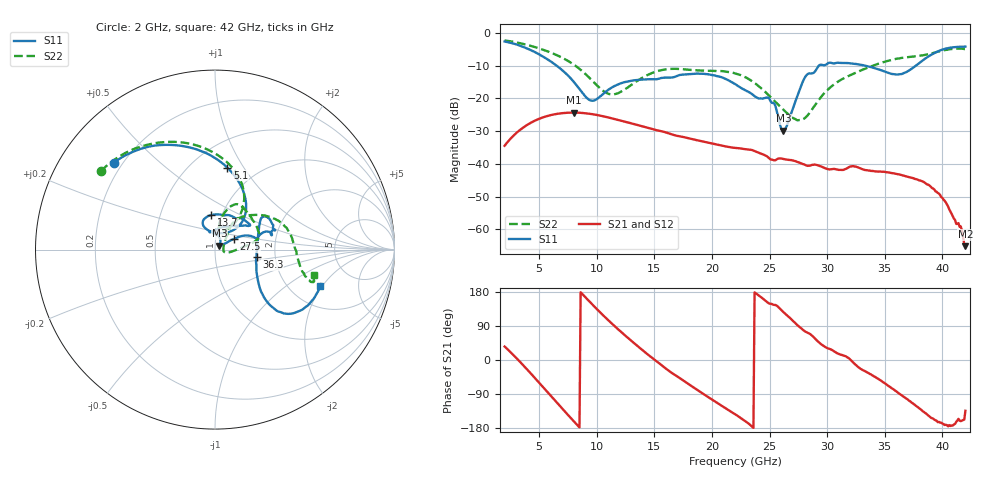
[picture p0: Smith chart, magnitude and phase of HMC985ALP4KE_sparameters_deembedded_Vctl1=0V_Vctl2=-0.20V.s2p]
!s2p File: Measurements: S11, S21, S12, S22
# GHz S dB R 50.0
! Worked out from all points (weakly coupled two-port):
!   401 points, 2 GHz to 42 GHz, reference 50 ohm
!   highest |S21| = -24.31 dB at 8 GHz (marker M1); lowest = -65.2 dB at 42 GHz (marker M2)
!   lowest |S11| = -29.8 dB at 26.2 GHz (marker M3), VSWR 1.07, Z = 52.5 + j2.21 ohm
!   |S11| at or under -10 dB: 6.529 GHz to 29.27 GHz (22.75 GHz wide, 127 % of centre); 33.34 GHz to 37.69 GHz (4.349 GHz wide, 12.2 % of centre)
!   |S22| runs from -26.7 to -2.3 dB; largest |S21 - S12| = 0.00014
!   S11 on the Smith chart (normalised r, x): 2 GHz: 0.17, +0.36; 5.1 GHz: 0.73, +0.85; 13.7 GHz: 0.89, +0.35; 27.5 GHz: 1.22, +0.15; 36.3 GHz: 1.60, -0.14; 42 GHz: 2.91, -1.91
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2  -2.57 139.4  -34.46 35.6  -34.48 35.6  -2.25 145.5
3.5  -4.07 111.5  -29.19 -10.1  -29.19 -10.1  -3.22 121.7
5.1  -6.71 81.5  -26.07 -63.4  -26.07 -63.5  -4.80 97.4
8  -14.89 44.9  -24.31 -161.6  -24.32 -161.6  -9.62 60.5
8.7  -18.05 51.5  -24.41 175.6  -24.42 175.6  -11.52 55.5
9.7  -20.68 87.2  -24.84 143.9  -24.84 143.9  -14.86 53.7
11.2  -16.89 115.8  -25.99 99.2  -25.99 99.2  -18.72 69.0
13.7  -14.29 96.7  -28.28 32.7  -28.28 32.7  -14.20 77.4
15.4  -13.94 73.0  -29.83 -8.1  -29.84 -8.1  -11.50 68.3
19.4  -12.51 34.7  -33.31 -92.5  -33.33 -92.4  -11.51 34.5
22  -15.57 52.2  -35.11 -142.8  -35.10 -142.7  -12.29 13.7
25  -20.23 97.6  -38.44 148.7  -38.44 148.8  -19.28 -2.8
26.2  -29.82 40.7  -38.49 126.4  -38.49 126.5  -23.44 -14.6
27.5  -18.42 29.5  -39.49 89.7  -39.51 90.0  -26.63 -2.3
28.1  -13.37 20.7  -40.34 75.1  -40.38 75.1  -25.90 19.8
28.7  -12.32 12.8  -40.28 64.0  -40.36 64.1  -23.29 37.7
31.1  -9.13 24.1  -41.83 15.1  -41.85 15.1  -14.49 55.8
35.4  -12.27 12.4  -42.64 -70.0  -42.69 -70.1  -8.40 25.9
36.3  -12.57 -10.1  -43.26 -89.6  -43.30 -89.5  -7.72 18.0
39.8  -5.31 -41.3  -49.49 -165.1  -49.54 -164.5  -5.51 -16.7
41.5  -4.18 -23.0  -59.26 -160.1  -59.31 -158.8  -4.74 -17.5
42  -4.14 -19.0  -65.17 -134.1  -66.66 -138.7  -4.89 -14.7
